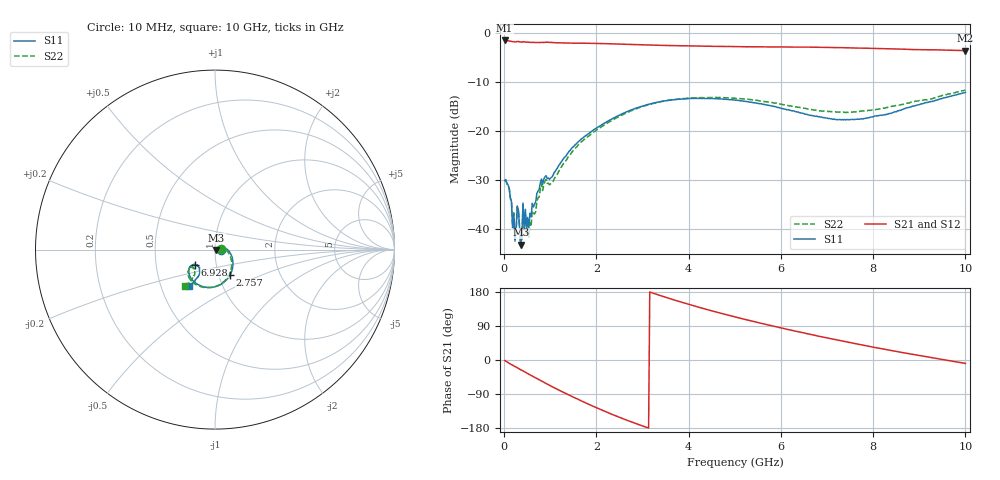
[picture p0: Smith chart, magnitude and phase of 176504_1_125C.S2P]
!  2-Port S-parameters saved by WinCal
! VAR MeasName=S-Parameters (CALIBRATED_DATA) read from VNA (N5242A)
! VAR MeasDate=2017-11-2 17:34:14
! VAR NAME=176504_1_125C
! VAR FILENAME=176504_1_125C.S2P
! VAR DATE=2017-11-2 17:34:14
! VAR PHYS_PORTS=2,3
# Hz S DB R 50
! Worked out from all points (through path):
!   401 points, 10 MHz to 10 GHz, reference 50 ohm
!   highest |S21| = -1.45 dB at 10 MHz (marker M1); lowest = -3.5 dB at 10 GHz (marker M2)
!   lowest |S11| = -43.1 dB at 359.6 MHz (marker M3), VSWR 1.01, Z = 50.7 - j0.138 ohm
!   |S11| at or under -10 dB: start of sweep to end of sweep
!   |S22| runs from -43.4 to -11.6 dB; largest |S21 - S12| = 0.013
!   S11 on the Smith chart (normalised r, x): 10 MHz: 1.07, +0.00; 2.757 GHz: 1.13, -0.33; 6.928 GHz: 0.79, -0.14; 10 GHz: 0.70, -0.30
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1e7  -30.01 0.8  -1.45 -1.1  -1.45 -1.1  -30.04 2.3
1.099e8  -31.61 -27.8  -1.55 -8.6  -1.55 -8.6  -31.73 -29.6
2.098e8  -36.85 -39.5  -1.68 -15.7  -1.68 -15.6  -36.63 -44.4
3.5965e8  -43.14 -11.2  -1.77 -25.8  -1.77 -25.8  -43.43 -29.5
3.84625e8  -40.98 21.7  -1.79 -27.2  -1.79 -27.2  -42.38 10.9
4.5955e8  -35.92 23.0  -1.77 -32.1  -1.77 -32.0  -37.03 16.1
4.84525e8  -39.64 23.9  -1.81 -34.1  -1.81 -34.1  -41.23 11.1
5.34475e8  -39.94 18.9  -1.81 -37.7  -1.81 -37.6  -41.60 3.6
8.34175e8  -30.84 23.1  -1.86 -57.0  -1.86 -56.9  -32.08 17.6
1.009e9  -29.51 13.4  -1.87 -68.5  -1.86 -68.4  -30.68 6.3
1.333675e9  -25.10 8.2  -1.98 -88.2  -1.97 -88.3  -26.06 4.0
1.683325e9  -21.48 -10.5  -2.02 -108.4  -2.01 -108.3  -22.06 -14.5
2.232775e9  -17.98 -37.2  -2.12 -138.1  -2.11 -138.0  -18.32 -39.9
2.75725e9  -15.62 -59.9  -2.27 -163.3  -2.27 -163.2  -15.80 -61.5
3.35665e9  -14.00 -82.9  -2.44 171.2  -2.45 171.3  -14.03 -84.0
4.180825e9  -13.29 -109.6  -2.60 140.6  -2.61 141.0  -13.13 -108.9
5.005e9  -13.61 -130.3  -2.70 113.7  -2.70 114.1  -13.27 -128.1
5.829175e9  -14.89 -143.4  -2.78 89.6  -2.82 90.1  -14.16 -140.2
6.678325e9  -16.79 -144.6  -2.82 66.6  -2.84 67.0  -15.58 -143.0
6.928075e9  -17.19 -142.7  -2.88 60.0  -2.88 60.5  -15.85 -142.4
8.35165e9  -16.35 -123.5  -3.14 26.0  -3.17 26.6  -15.05 -129.4
1e10  -12.06 -124.9  -3.53 -9.0  -3.54 -8.2  -11.57 -129.9
